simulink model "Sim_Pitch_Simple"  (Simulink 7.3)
settings: Solver=ode23s  StartTime=0.0  StopTime=20  RelTol=1e-3
InitFcn:
  | init
StartFcn:
  | init
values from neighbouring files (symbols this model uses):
  d2r = pi/180    (= 0.0174532925199)    [init.m]    (also in robust.m)
  r2d = 180/pi    (= 57.2957795131)    [init.m]    (also in robust.m)
undefined symbols (not defined in the file or in its folder): Aps, Bps, Cps, Dps, Kmix, Kq

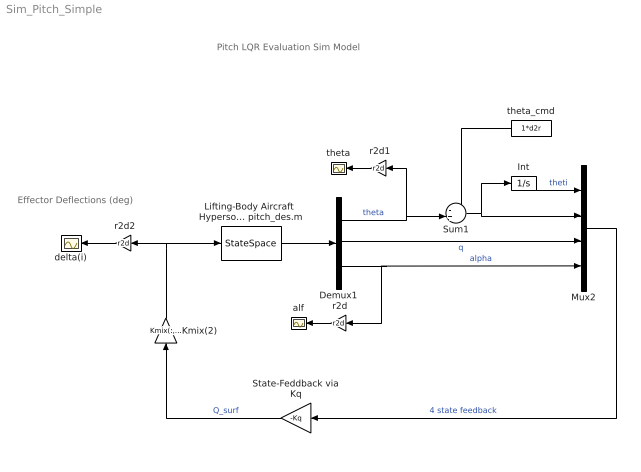
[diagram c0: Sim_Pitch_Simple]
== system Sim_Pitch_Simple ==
  note: Effector Deflections (deg)
  note: Pitch LQR Evaluation Sim Model
  " r2d" : Gain  Gain=r2d  ParameterDataType=sfix(16)  ParameterScaling=2^0  OutDataType=sfix(16)  OutScaling=2^0
  " r2d1" : Gain  Gain=r2d  ParameterDataType=sfix(16)  ParameterScaling=2^0  OutDataType=sfix(16)  OutScaling=2^0
  " r2d2" : Gain  Gain=r2d  ParameterDataType=sfix(16)  ParameterScaling=2^0  OutDataType=sfix(16)  OutScaling=2^0
  Demux1 : Demux  Outputs=3
  Int : Integrator
  Kmix(2) : Gain  Gain=Kmix(:,2)  Multiplication=Matrix(K*u)  ParameterDataType=sfix(16)  ParameterScaling=2^0  OutDataType=sfix(16)  OutScaling=2^0
  Lifting-Body Aircraft  Hypersonic Pitch  Design Model from file pitch_des.m : StateSpace  A=Aps  B=Bps  C=Cps  D=Dps
  Mux2 : Mux
  State-Feddback via Kq : Gain  Gain=-Kq  Multiplication=Matrix(K*u)  ParameterDataType=sfix(16)  ParameterScaling=2^0  OutDataType=sfix(16)  OutScaling=2^0
  Sum1 : Sum  Inputs=-+|  OutDataType=sfix(16)  OutScaling=2^0
  alf : Scope
  delta(i) : Scope
  theta : Scope
  theta_cmd : Constant  Value=1*d2r  OutDataType=sfix(16)  OutScaling=2^0
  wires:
  Demux1/2 -> Mux2/3  "q"
  Mux2/1 -> State-Feddback via Kq/1  "4 state feedback"
  State-Feddback via Kq/1 -> Kmix(2)/1  "Q_surf"
  " r2d"/1 -> alf/1
  Lifting-Body Aircraft  Hypersonic Pitch  Design Model from file pitch_des.m/1 -> Demux1/1
  Demux1/3 -> " r2d"/1, Mux2/4  "alpha"
  Demux1/1 -> " r2d1"/1, Sum1/2  "theta"
  " r2d1"/1 -> theta/1
  Kmix(2)/1 -> Lifting-Body Aircraft  Hypersonic Pitch  Design Model from file pitch_des.m/1, " r2d2"/1
  " r2d2"/1 -> delta(i)/1
  Int/1 -> Mux2/1  "theti"
  Sum1/1 -> Mux2/2, Int/1
  theta_cmd/1 -> Sum1/1
